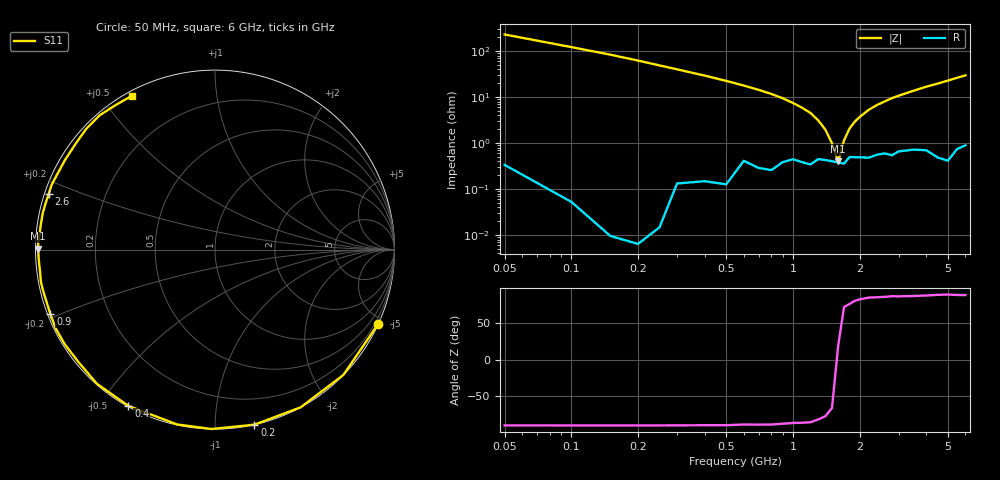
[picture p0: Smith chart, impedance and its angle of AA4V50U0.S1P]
! Infineon Technologies  Discrete & RF Semiconductors
! BBY66-02W
! Si Tuning Diode in SCD-80
! VR = 4.5 V
! S-Parameters:  June  2000
# GHz  S  MA  R  50
!  f  S11
! GHz  MAG  ANG
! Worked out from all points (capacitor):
!   34 points, 50 MHz to 6 GHz, reference 50 ohm
!   read as one part to ground: C = 12.9 pF near 50 MHz
!   lowest |Z| = 402 mohm at 1.6 GHz (marker M1)
!   series resonance near 1.588 GHz, so ESL is about 780 pH
!   S11 on the Smith chart (normalised r, x): 50 MHz: 0.01, -4.63; 200 MHz: 0.00, -1.25; 400 MHz: 0.00, -0.59; 900 MHz: 0.01, -0.19; 2.6 GHz: 0.01, +0.16; 6 GHz: 0.02, +0.59
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0.05  0.9994 -24.4
0.1  0.9997 -44.3
0.15  0.9999 -61.5
0.2  0.9999 -77.3
0.25  0.9997 -91.1
0.3  0.9968 -102.2
0.4  0.9956 -119.0
0.5  0.9958 -131.4
0.6  0.9855 -140.6
0.7  0.9894 -147.8
0.8  0.9902 -153.6
0.9  0.9852 -158.6
1  0.9827 -163.0
1.2  0.9865 -169.7
1.3  0.9822 -172.9
1.4  0.983 -175.6
1.6  0.9849 179.7
1.9  0.9805 173.4
2.2  0.9811 167.9
2.4  0.9782 164.6
2.6  0.977 161.6
2.8  0.9792 158.4
3.5  0.9735 149.2
4  0.9752 142.6
4.5  0.9833 136.9
5  0.9864 130.7
5.5  0.9771 124.4
6  0.9738 118.5
